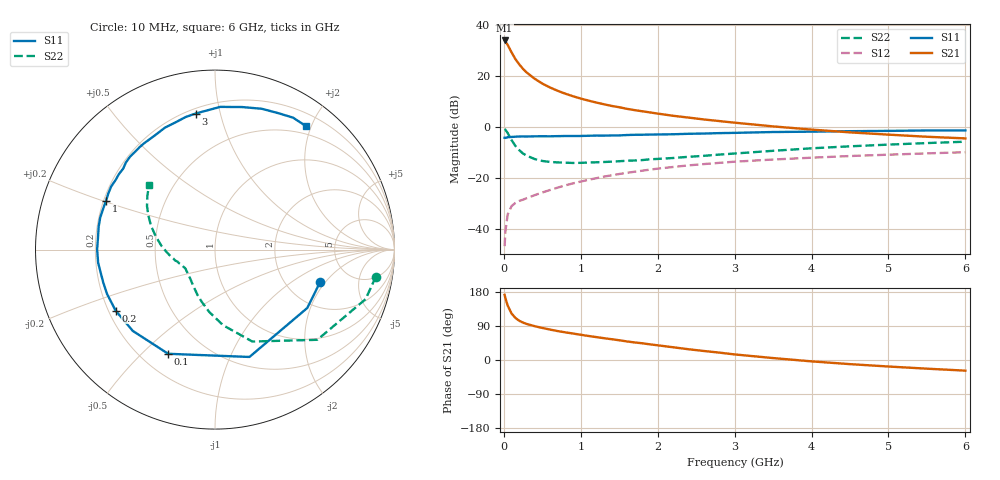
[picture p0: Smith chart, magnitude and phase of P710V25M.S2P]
! SIEMENS Small Signal Semiconductors
! BFP196
! Si NPN RF Bipolar Junction Transistor in SOT143
! VCE = 10 V  IC = 25 mA
! Common Emitter S-Parameters:  May  1996
# GHz  S  MA  R  50
!  f  S11  S21  S12  S22
! GHz  MAG  ANG  MAG  ANG  MAG  ANG  MAG  ANG
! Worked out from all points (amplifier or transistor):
!   36 points, 10 MHz to 6 GHz, reference 50 ohm
!   highest |S21| = 34.1 dB at 10 MHz (marker M1)
!   |S21| within 3 dB of that: start of sweep to 71.49 MHz
!   unconditionally stable (mu >= 1): 679.7 MHz to 4.309 GHz
!   at 250 MHz: K = 0.62, MSG = 25.7 dB, |S12| = -28.6 dB
!   at 1.4 GHz: K = 1.10, MAG = 11.7 dB, |S12| = -19.0 dB
!   at 6 GHz: K = 0.96, MSG = 2.7 dB, |S12| = -9.9 dB
!   S11 on the Smith chart (normalised r, x): 10 MHz: 3.07, -1.76; 100 MHz: 0.31, -0.60; 200 MHz: 0.23, -0.27; 1 GHz: 0.21, +0.20; 3 GHz: 0.23, +0.84; 6 GHz: 0.38, +1.92
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0.01  0.6132 -17.0  50.54 171.8  0.0045 77.4  0.909 -9.5
0.02  0.6084 -32.3  48.11 163.2  0.0087 72.0  0.8834 -18.2
0.05  0.6282 -72.2  41.35 143.7  0.019 59.5  0.7599 -41.4
0.1  0.6364 -114.2  29.53 122.8  0.0277 46.8  0.5528 -67.9
0.15  0.6442 -135.3  21.75 111.1  0.0319 42.3  0.4244 -83.8
0.2  0.6497 -148.4  17.12 103.6  0.035 41.6  0.3495 -95.2
0.25  0.6504 -157.7  13.89 98.6  0.0371 42.4  0.2999 -104.3
0.3  0.6491 -163.7  11.71 94.9  0.0398 43.7  0.2712 -111.0
0.4  0.6553 -173.6  8.926 89.3  0.0454 46.6  0.2339 -121.6
0.5  0.6567 179.9  7.162 84.6  0.0513 49.4  0.2143 -129.5
0.6  0.6554 173.9  5.994 80.3  0.0574 51.3  0.2052 -135.6
0.7  0.6607 168.8  5.157 76.3  0.064 52.2  0.2005 -139.9
0.8  0.6639 164.4  4.517 73.0  0.0709 52.6  0.198 -143.6
1  0.6652 156.0  3.629 66.6  0.0842 53.5  0.1967 -148.9
1.1  0.6716 152.2  3.306 63.4  0.091 53.2  0.1997 -151.1
1.6  0.6945 135.6  2.277 49.0  0.1252 49.9  0.2163 -160.4
2.2  0.7187 117.9  1.661 33.6  0.1631 43.3  0.245 -169.9
3  0.7658 98.1  1.216 14.7  0.2072 33.2  0.3003 175.7
3.5  0.7957 87.9  1.027 5.1  0.2288 26.8  0.3395 167.1
4.5  0.8268 71.6  0.783 -10.9  0.268 15.6  0.4163 153.0
5.5  0.8541 59.4  0.642 -22.9  0.3023 5.2  0.4823 141.4
6  0.8546 53.7  0.596 -28.1  0.3184 -0.4  0.5131 135.7
